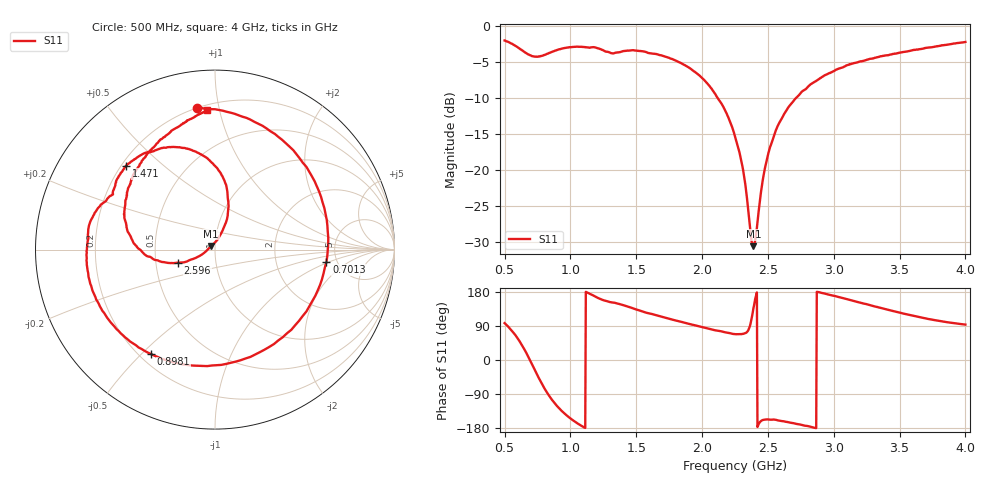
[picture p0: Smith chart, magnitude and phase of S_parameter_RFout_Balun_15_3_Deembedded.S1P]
!Agilent Technologies,E5071B,MY42403504,A.06.51
!Date: Wed Feb 26 14:58:38 2014
!Data & Calibration Information:
!Freq	S11:SOLT1(ON)
# Hz S dB R 50
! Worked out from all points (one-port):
!   801 points, 500 MHz to 4 GHz, reference 50 ohm
!   lowest |S11| = -30.6 dB at 2.39 GHz (marker M1), VSWR 1.06, Z = 47.9 + j1.94 ohm
!   |S11| at or under -10 dB: 2.118 GHz to 2.713 GHz (594.1 MHz wide, 24.6 % of centre)
!   S11 on the Smith chart (normalised r, x): 500 MHz: 0.20, +0.86; 701.2 MHz: 4.11, -0.91; 898.1 MHz: 0.25, -0.53; 1.471 GHz: 0.22, +0.38; 2.596 GHz: 0.65, -0.10; 4 GHz: 0.23, +0.91
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5e8  -1.98 97.3
5.525e8  -2.43 78.4
5.9625e8  -2.89 58.5
6.53125e8  -3.62 26.2
7.0125e8  -4.09 -6.2
7.5375e8  -4.24 -43.3
7.975e8  -4.02 -71.7
8.4125e8  -3.72 -96.1
8.98125e8  -3.32 -121.5
9.375e8  -3.10 -135.7
1.0075e9  -2.91 -156.1
1.08625e9  -2.88 -174.2
1.22625e9  -3.18 161.1
1.375e9  -3.61 147.5
1.47125e9  -3.33 136.7
1.655e9  -3.89 117.8
1.8125e9  -4.89 103.1
2.061875e9  -8.47 81.3
2.25e9  -15.33 68.2
2.31125e9  -19.99 68.9
2.3725e9  -29.47 103.4
2.39e9  -30.63 136.6
2.48625e9  -19.03 -156.8
2.595625e9  -13.16 -160.7
2.6875e9  -10.57 -166.4
3.125e9  -5.29 158.3
3.5625e9  -3.50 119.9
4e9  -2.19 93.4
